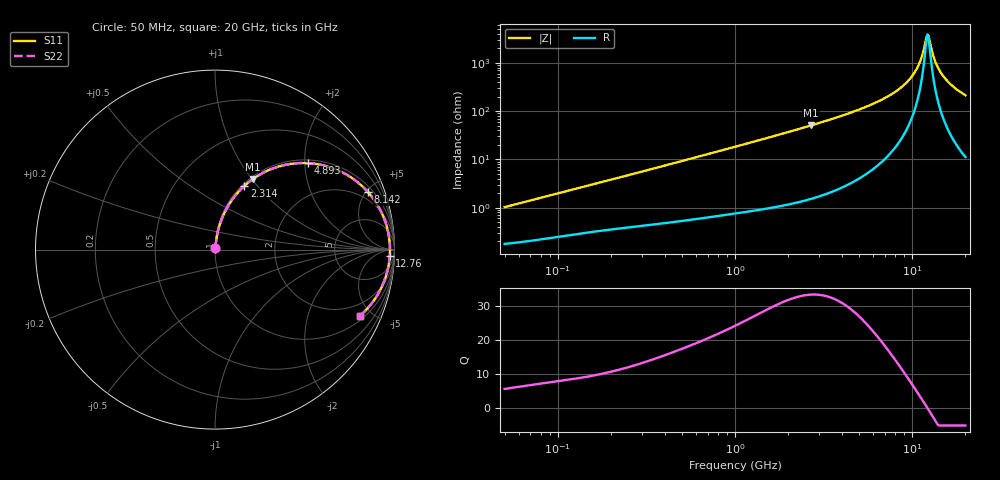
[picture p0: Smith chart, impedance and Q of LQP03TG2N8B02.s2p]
!Murata Part Number: LQP03TG2N8B02
!These Parameters are Measured in Series Mode Connection
!  o--[Z]--o
!Port1  Port2
!  o-------o
!Freq. Start=50[MHz] Stop=20[GHz], 401[Steps]
# Hz S RI R 50
!Freq.(Hz) S11(Real) S11(Imag) S21(Real) S21(Imag) S12(Real) S12(Imag) S22(Real) S22(Imag)
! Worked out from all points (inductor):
!   401 points, 50 MHz to 20 GHz, reference 50 ohm
!   read as one part in series: L = 3.19 nH near 51.52 MHz
!   highest Q = 33.3 at 2.687 GHz (marker M1), where L = 2.99 nH
!   self-resonance near 12.2 GHz
!   S11 on the Smith chart (normalised r, x): 50 MHz: 1.00, +0.02; 2.314 GHz: 1.03, +0.86; 4.893 GHz: 1.08, +2.08; 8.142 GHz: 1.38, +5.18; 12.76 GHz: 26, -36; 20 GHz: 1.22, -4.27
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5e7  0.00187 0.0101  0.9981 -0.0101  0.9981 -0.0101  0.00187 0.0101
1.364002e8  0.00361 0.0262  0.9964 -0.0262  0.9964 -0.0262  0.00361 0.0262
3.721004e8  0.00926 0.068  0.9907 -0.068  0.9907 -0.068  0.00926 0.068
1e9  0.0389 0.1737  0.9611 -0.1737  0.9611 -0.1737  0.0389 0.1737
2.313601e9  0.1633 0.3547  0.8367 -0.3547  0.8367 -0.3547  0.1633 0.3547
2.687447e9  0.2103 0.3928  0.7897 -0.3928  0.7897 -0.3928  0.2103 0.3928
2.728004e9  0.2156 0.3965  0.7844 -0.3965  0.7844 -0.3965  0.2156 0.3965
4.89267e9  0.5185 0.4818  0.4815 -0.4818  0.4815 -0.4818  0.5185 0.4818
6.034176e9  0.6621 0.4513  0.3379 -0.4513  0.3379 -0.4513  0.6621 0.4513
7.442007e9  0.8014 0.3699  0.1986 -0.3699  0.1986 -0.3699  0.8014 0.3699
8.141811e9  0.8537 0.3189  0.1463 -0.3189  0.1463 -0.3189  0.8537 0.3189
9.316812e9  0.9179 0.2264  0.0821 -0.2264  0.0821 -0.2264  0.9179 0.2264
1.034674e10  0.9526 0.1438  0.0474 -0.1438  0.0474 -0.1438  0.9526 0.1438
1.115139e10  0.9679 0.0809  0.0321 -0.0809  0.0321 -0.0809  0.9679 0.0809
1.183995e10  0.974 0.0293  0.026 -0.0293  0.026 -0.0293  0.974 0.0293
1.220001e10  0.975 0.00323  0.025 -0.00323  0.025 -0.00323  0.975 0.00323
1.238412e10  0.975 -0.0098  0.025 0.0098  0.025 0.0098  0.975 -0.0098
1.276073e10  0.9738 -0.0358  0.0262 0.0358  0.0262 0.0358  0.9738 -0.0358
1.354865e10  0.9674 -0.0875  0.0326 0.0875  0.0326 0.0875  0.9674 -0.0875
1.482269e10  0.9476 -0.1626  0.0524 0.1626  0.0524 0.1626  0.9476 -0.1626
1.696185e10  0.8971 -0.2658  0.1029 0.2658  0.1029 0.2658  0.8971 -0.2658
2e10  0.8079 -0.3686  0.1921 0.3686  0.1921 0.3686  0.8079 -0.3686
